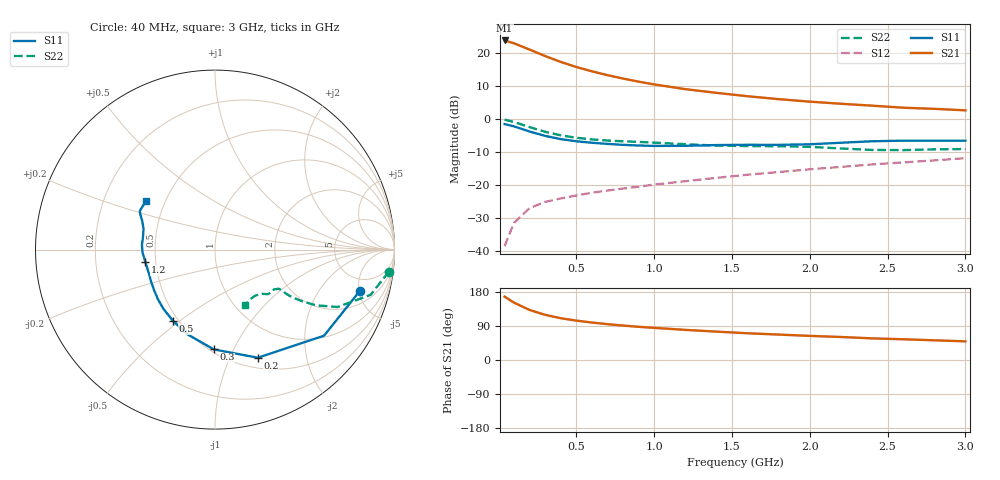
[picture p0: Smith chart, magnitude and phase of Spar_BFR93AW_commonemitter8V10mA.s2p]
! Filename:  BFR93AWF.S2P  Version:  4.0
! NXP part #: BFR93AW  Date: Jun 1994
! Bias condition: Vce=8V, Ic=10mA
#  MHz  S  MA  R  50
! Freq  S11  S21  S12  S22  !GUM [dB]
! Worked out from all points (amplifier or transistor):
!   21 points, 40 MHz to 3 GHz, reference 50 ohm
!   highest |S21| = 23.7 dB at 40 MHz (marker M1)
!   |S21| within 3 dB of that: start of sweep to 212.8 MHz
!   unconditionally stable (mu >= 1): 960.8 MHz to end of sweep
!   at 300 MHz: K = 0.51, MSG = 22.0 dB, |S12| = -25.0 dB
!   at 1 GHz: K = 1.02, MAG = 14.4 dB, |S12| = -19.8 dB
!   at 3 GHz: K = 1.03, MAG = 6.1 dB, |S12| = -11.8 dB
!   lowest NFmin = 1.40 dB at 500 MHz
!   S11 on the Smith chart (normalised r, x): 40 MHz: 3.24, -5.05; 200 MHz: 0.62, -1.28; 300 MHz: 0.52, -0.84; 500 MHz: 0.47, -0.47; 1.2 GHz: 0.44, -0.07; 3 GHz: 0.39, +0.27
40  0.838 -16.1  15.37 167.2  0.012 81.6  0.977 -7.2
100  0.774 -38.3  13.93 151.4  0.027 70.6  0.903 -16.2
200  0.648 -68.4  11.2 132.1  0.045 60.2  0.754 -25.1
300  0.556 -90.7  8.936 119.2  0.056 55.0  0.642 -28.9
400  0.497 -107.7  7.291 110.3  0.063 53.6  0.568 -30.6
500  0.461 -120.4  6.109 104.0  0.07 54.1  0.521 -31.4
600  0.438 -130.9  5.255 98.9  0.077 55.4  0.492 -31.8
700  0.421 -139.3  4.599 94.6  0.083 56.9  0.473 -31.8
800  0.407 -146.7  4.087 90.9  0.089 58.4  0.461 -31.8
900  0.398 -153.4  3.669 87.6  0.095 60.1  0.451 -31.5
1000  0.392 -159.5  3.333 84.8  0.102 61.4  0.44 -31.2
1200  0.394 -169.9  2.827 79.5  0.115 64.0  0.416 -31.6
1400  0.404 -177.6  2.485 74.9  0.129 66.1  0.397 -33.9
1600  0.408 176.3  2.209 70.6  0.144 67.5  0.39 -37.4
1800  0.407 170.3  1.996 67.1  0.158 69.3  0.388 -39.5
2000  0.415 163.7  1.829 63.6  0.174 70.6  0.38 -40.8
2200  0.438 158.1  1.7 60.7  0.189 71.7  0.359 -43.3
2400  0.461 154.6  1.591 57.1  0.206 72.4  0.341 -48.5
2600  0.471 152.8  1.482 54.7  0.221 72.6  0.339 -55.0
2800  0.47 149.5  1.424 52.0  0.237 73.4  0.348 -59.3
3000  0.47 145.0  1.352 49.2  0.256 73.7  0.352 -62.0
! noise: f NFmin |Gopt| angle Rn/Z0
500  1.4  0.259  44  0.167
1000  2  0.234  136.2  0.218
2000  3  0.566  -154.8  0.14
